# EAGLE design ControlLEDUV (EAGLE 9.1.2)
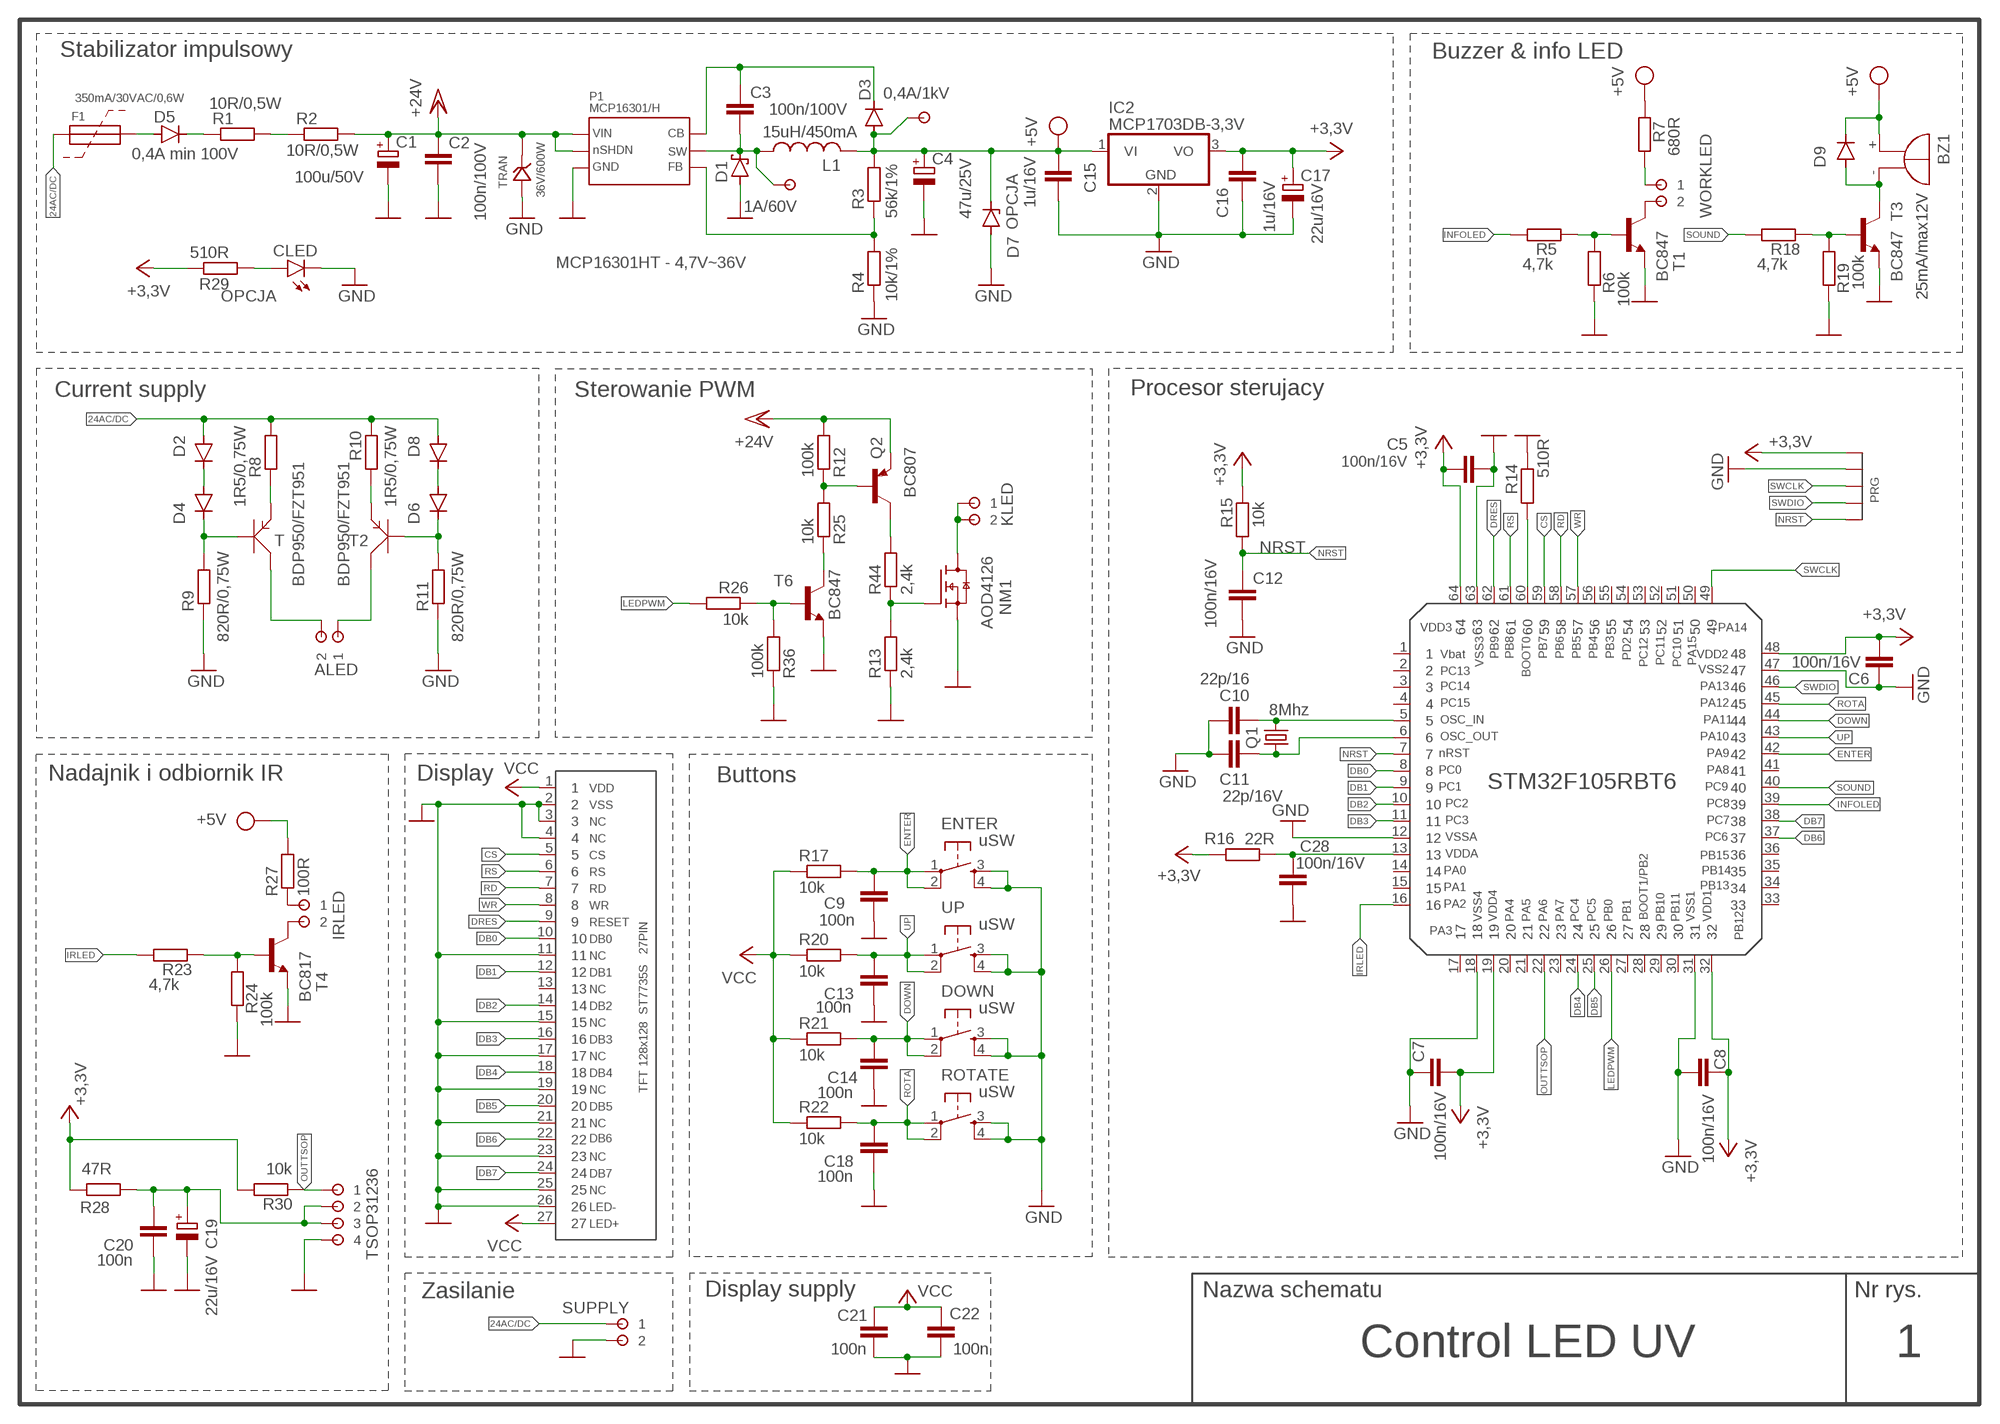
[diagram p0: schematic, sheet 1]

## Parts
ALED  ARK254  [ARK254]
BZ1  25mA/max12V  F/TMB  [F/TMB]
C1  100u/50V  CPOL-EU175TMP-0810  [175TMP-0810]
C2  100n/100V  C-EUC1206  [C1206]
C3  100n/100V  C-EUC0805  [C0805]
C4  47u/25V  CPOL-EU153CLV-0605  [153CLV-0605]
C5  100n/16V  C-EUC0805  [C0805]
C6  100n/16V  C-EUC0805  [C0805]
C7  100n/16V  C-EUC0805  [C0805]
C8  100n/16V  C-EUC0805  [C0805]
C9  100n  C-EUC0805  [C0805]
C10  22p/16  C-EUC0805  [C0805]
C11  22p/16V  C-EUC0805  [C0805]
C12  100n/16V  C-EUC0805  [C0805]
C13  100n  C-EUC0805  [C0805]
C14  100n  C-EUC0805  [C0805]
C15  1u/16V  C-EUC0805  [C0805]
C16  1u/16V  C-EUC0805  [C0805]
C17  22u/16V  CPOL-EU153CLV-0505  [153CLV-0505]
C18  100n  C-EUC0805  [C0805]
C19  22u/16V  CPOL-EU153CLV-0505  [153CLV-0505]
C20  100n  C-EUC0805  [C0805]
C21  100n  C-EUC0805  [C0805]
C22  100n  C-EUC0805  [C0805]
C28  100n/16V  C-EUC0805  [C0805]
CLED  LEDCHIPLED_0805  [CHIPLED_0805]
D1  1A/60V  SCHOTTKY-DIODESMD  [SMB]
D2  DIODE-MINIMELF  [MINIMELF]
D3  0,4A/1kV  DIODE-MINIMELF  [MINIMELF]
D4  DIODE-MINIMELF  [MINIMELF]
D5  0,4A min 100V  DIODE-MINIMELF  [MINIMELF]
D6  DIODE-MINIMELF  [MINIMELF]
D7  ZENER-DIODESOD80C  [SOD80C]
D8  DIODE-MINIMELF  [MINIMELF]
D9  DIODE-MINIMELF  [MINIMELF]
DOWN  uSW  DTSM-6  [DTSM-6]
ENTER  uSW  DTSM-6  [DTSM-6]
F1  350mA/30VAC/0,6W  FUSE1  [FUSE1]
IC2  MCP1703DB-3,3V  MCP1703DB  [SOT223]
IRLED  ARK254  [ARK254]
KLED  ARK254  [ARK254]
L1  15uH/450mA  L-USL4532P  [L4532P]
NM1  AOD4126  [AOD4126]
P1  MCP16301/H  MCP16301  [MCP16301]
PRG  GOLDPIN5  [GOLDPIN5]
Q1  8Mhz  CRYSTALHC49S  [HC49/S]
Q2  BC807  BC807-16LT1SMD  [SOT23-BEC]
R1  10R/0,5W  R-EU_M1206  [M1206]
R2  10R/0,5W  R-EU_M1206  [M1206]
R3  56k/1%  R-EU_R0805  [R0805]
R4  10k/1%  R-EU_R0805  [R0805]
R5  4,7k  R-EU_R0805  [R0805]
R6  100k  R-EU_R0805  [R0805]
R7  680R  R-EU_R0805  [R0805]
R8  1R5/0,75W  R-EU_R2010  [R2010]
R9  820R/0,75W  R-EU_R2010  [R2010]
R10  1R5/0,75W  R-EU_R2010  [R2010]
R11  820R/0,75W  R-EU_R2010  [R2010]
R12  100k  R-EU_R0805  [R0805]
R13  2,4k  R-EU_R0805  [R0805]
R14  510R  R-EU_R0805  [R0805]
R15  10k  R-EU_R0805  [R0805]
R16  22R  R-EU_R0805  [R0805]
R17  10k  R-EU_R0805  [R0805]
R18  4,7k  R-EU_R0805  [R0805]
R19  100k  R-EU_R0805  [R0805]
R20  10k  R-EU_R0805  [R0805]
R21  10k  R-EU_R0805  [R0805]
R22  10k  R-EU_R0805  [R0805]
R23  4,7k  R-EU_R0805  [R0805]
R24  100k  R-EU_R0805  [R0805]
R25  10k  R-EU_R0805  [R0805]
R26  10k  R-EU_R0805  [R0805]
R27  100R  R-EU_M1206  [M1206]
R28  47R  R-EU_R0805  [R0805]
R29  510R  R-EU_R0805  [R0805]
R30  10k  R-EU_R0805  [R0805]
R36  100k  R-EU_R0805  [R0805]
R44  2,4k  R-EU_R0805  [R0805]
ROTATE  uSW  DTSM-6  [DTSM-6]
SUPPLY  ARK254  [ARK254]
T  BDP950/FZT951  BDP950  [FZT951]
T1  BC847  [SOT23]
T2  BDP950/FZT951  BDP950  [FZT951]
T3  BC847  [SOT23]
T4  BC817  BC847  [SOT23]
T6  BC847  [SOT23]
TRAN  36V/600W  TRANSIL2  [DO214AC_BIG]
TSOP31236  ARK254-4  [ARK254-4]
U$3  STM32F105RBT6  [STM32F105RBT6]
U$4  TFT128128  [TFT128128]
U$5  PAD5  [PAD5]
U$6  PAD5  [PAD5]
UP  uSW  DTSM-6  [DTSM-6]
WORKLED  ARK254  [ARK254]

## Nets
24AC/DC: D2.A D8.A F1.1 R8.2 R10.2 SUPPLY.1
CS: U$3.59 U$4.5
DB0: U$3.8 U$4.10
DB1: U$3.9 U$4.12
DB2: U$3.10 U$4.14
DB3: U$3.11 U$4.16
DB4: U$3.24 U$4.18
DB5: U$3.25 U$4.20
DB6: U$3.37 U$4.22
DB7: U$3.38 U$4.24
DOWN: C14.1 DOWN.1 DOWN.2 R21.2 U$3.44
DRES: U$3.62 U$4.9
ENTER: C9.1 ENTER.1 ENTER.2 R17.2 U$3.42
GND: C1.- C2.2 C4.- C5.1 C6.1 C7.1 C8.2 C9.2 C10.1 C11.1 C12.2 C13.2 C14.2 C15.2 C16.2 C17.- C18.2 C19.- C20.2 C21.2 C22.2 C28.1 CLED.C D1.A D7.A DOWN.3 DOWN.4 ENTER.3 ENTER.4 IC2.2(GND) NM1.S P1.2 PRG.2 R4.1 R6.1 R9.1 R11.1 R13.1 R14.2 R19.1 R24.1 R36.1 ROTATE.3 ROTATE.4 SUPPLY.2 T1.2(E) T3.2(E) T4.2(E) T6.2(E) TRAN.P$1 TSOP31236.4 U$3.12 U$3.18 U$3.31 U$3.47 U$3.63 U$4.2 U$4.3 U$4.4 U$4.11 U$4.15 U$4.17 U$4.19 U$4.21 U$4.23 U$4.25 U$4.26 UP.3 UP.4
INFOLED: R5.1 U$3.39
IRLED: R23.1 U$3.16
LAMP1_PWM: Q2.C R44.2
LEDPWM: R26.2 U$3.26
N$1: D5.C R1.1
N$2: R1.2 R2.1
N$3: R5.2 R6.2 T1.1(B)
N$4: T1.3(C) WORKLED.2
N$5: C3.1 D3.C P1.1
N$6: C3.2 D1.C L1.1 P1.6 U$5.1
N$7: P1.3 R3.1 R4.2
N$8: R7.1 WORKLED.1
N$9: D5.A F1.2
N$10: KLED.1 KLED.2 NM1.D
N$11: R8.1 T.3
N$12: ALED.2 T.2 T.4
N$13: D2.C D4.A
N$14: D4.C R9.2 T.1
N$15: ALED.1 T2.2 T2.4
N$16: R10.1 T2.3
N$17: D6.C R11.2 T2.1
N$18: D6.A D8.C
N$19: NM1.G R13.2 R44.1
N$20: C10.2 Q1.2 U$3.5
N$21: C11.2 Q1.1 U$3.6
N$22: R18.2 R19.2 T3.1(B)
N$23: R14.1 U$3.60
N$24: BZ1.- D9.A T3.3(C)
N$25: C28.2 R16.1 U$3.13
N$26: R23.2 R24.2 T4.1(B)
N$27: IRLED.2 T4.3(C)
N$28: Q2.B R12.1 R25.2
N$29: R25.1 T6.3(C)
N$30: R26.1 R36.2 T6.1(B)
N$31: IRLED.1 R27.1
N$32: CLED.A R29.1
N$34: C19.+ C20.1 R28.2 TSOP31236.2 TSOP31236.3
NRST: C12.1 PRG.5 R15.1 U$3.7
OUTTSOP: R30.2 TSOP31236.1 U$3.22
RD: U$3.58 U$4.7
ROTA: C18.1 R22.2 ROTATE.1 ROTATE.2 U$3.45
RS: U$3.61 U$4.6
SOUND: R18.1 U$3.40
SWCLK: PRG.3 U$3.49
SWDIO: PRG.4 U$3.46
UP: C13.1 R20.2 U$3.43 UP.1 UP.2
VCC: C5.2 C6.2 C7.2 C8.1 C16.1 C17.+ C21.1 C22.1 IC2.3(VO) PRG.1 R15.2 R16.2 R17.1 R20.1 R21.1 R22.1 R28.1 R29.2 R30.1 U$3.19 U$3.32 U$3.48 U$3.64 U$4.1 U$4.27 ; supply symbol labelled +3,3V
VCC/2: C1.+ C2.1 P1.4 P1.5 Q2.E R2.2 R12.2 TRAN.P$2 ; supply symbol labelled +24V
VDD: BZ1.+ C4.+ C15.1 D3.A D7.C D9.C IC2.1(VI) L1.2 R3.2 R7.2 R27.2 U$6.1 ; supply symbol labelled +5V
WR: U$3.57 U$4.8
Unconnected: U$3.1 U$3.2 U$3.3 U$3.4 U$3.14 U$3.15 U$3.17 U$3.20 U$3.21 U$3.23 U$3.27 U$3.28 U$3.29 U$3.30 U$3.33 U$3.34 U$3.35 U$3.36 U$3.41 U$3.50 U$3.51 U$3.52 U$3.53 U$3.54 U$3.55 U$3.56 U$4.13

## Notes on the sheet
- Stabilizator impulsowy | Buzzer & info LED
- OPCJA
- MCP16301HT - 4,7V~36V
- OPCJA
- Current supply | Sterowanie PWM | Procesor sterujacy
- Nadajnik i odbiornik IR | Display | Buttons
- Zasilanie | Display supply
- Control LED UV | 1

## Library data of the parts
ALED IRLED KLED SUPPLY WORKLED = ark254:ARK254
BZ1 = buzzer:F/TMB: BUZZER; OC_FARNELL: unknown; OC_NEWARK: unknown
C1 C4 C17 C19 = rcl:CPOL-EU: POLARIZED CAPACITOR, European symbol; SPICEPREFIX: C
C2 C3 C5-C16 C18 C20-C22 C28 = rcl:C-EU: CAPACITOR, European symbol; SPICEPREFIX: C
CLED = led:LED: LED
D1 = diode:SCHOTTKY-DIODE: Schottky Diode
D2-D6 D8 D9 = diode:DIODE-: DIODE
D7 = diode:ZENER-DIODE: Z-Diode
DOWN ENTER ROTATE UP = switch-tact:DTSM-6
F1 = Fuse:FUSE1
IC2 = linear:MCP1703: 250 mA, 16V, Low Quiescent Current LDO Regulator Source: http://ww1.microchip.com/downloads/en/DeviceDoc/22049b.pdf
L1 = rcl:L-US: INDUCTOR, American symbol; SPICEPREFIX: L
NM1 = AOD4126:AOD4126
P1 = Regulatory:MCP16301
PRG = Goldpin5:GOLDPIN5: 3 Goldpin
Q1 = crystal:CRYSTAL: CRYSTAL; OC_FARNELL: 1667008; OC_NEWARK: unknown
Q2 = transistor-pnp:BC807*: PNP Transistror
R1-R30 R36 R44 = rcl:R-EU_: RESISTOR, European symbol; SPICEPREFIX: R
T T2 = transistorpnp:BDP950
T1 T3 T4 = transistor-neu-to92:BC847: NPN TRANSISTOR
T6 = transistor:BC847: NPN TRANSISTOR; SPICEPREFIX: J
TRAN = transil2:TRANSIL2
TSOP31236 = ark254:ARK254-4
U$3 = STM32F105RBT6:STM32F105RBT6
U$4 = tft128128:TFT128128
U$5 U$6 = PAD:PAD5

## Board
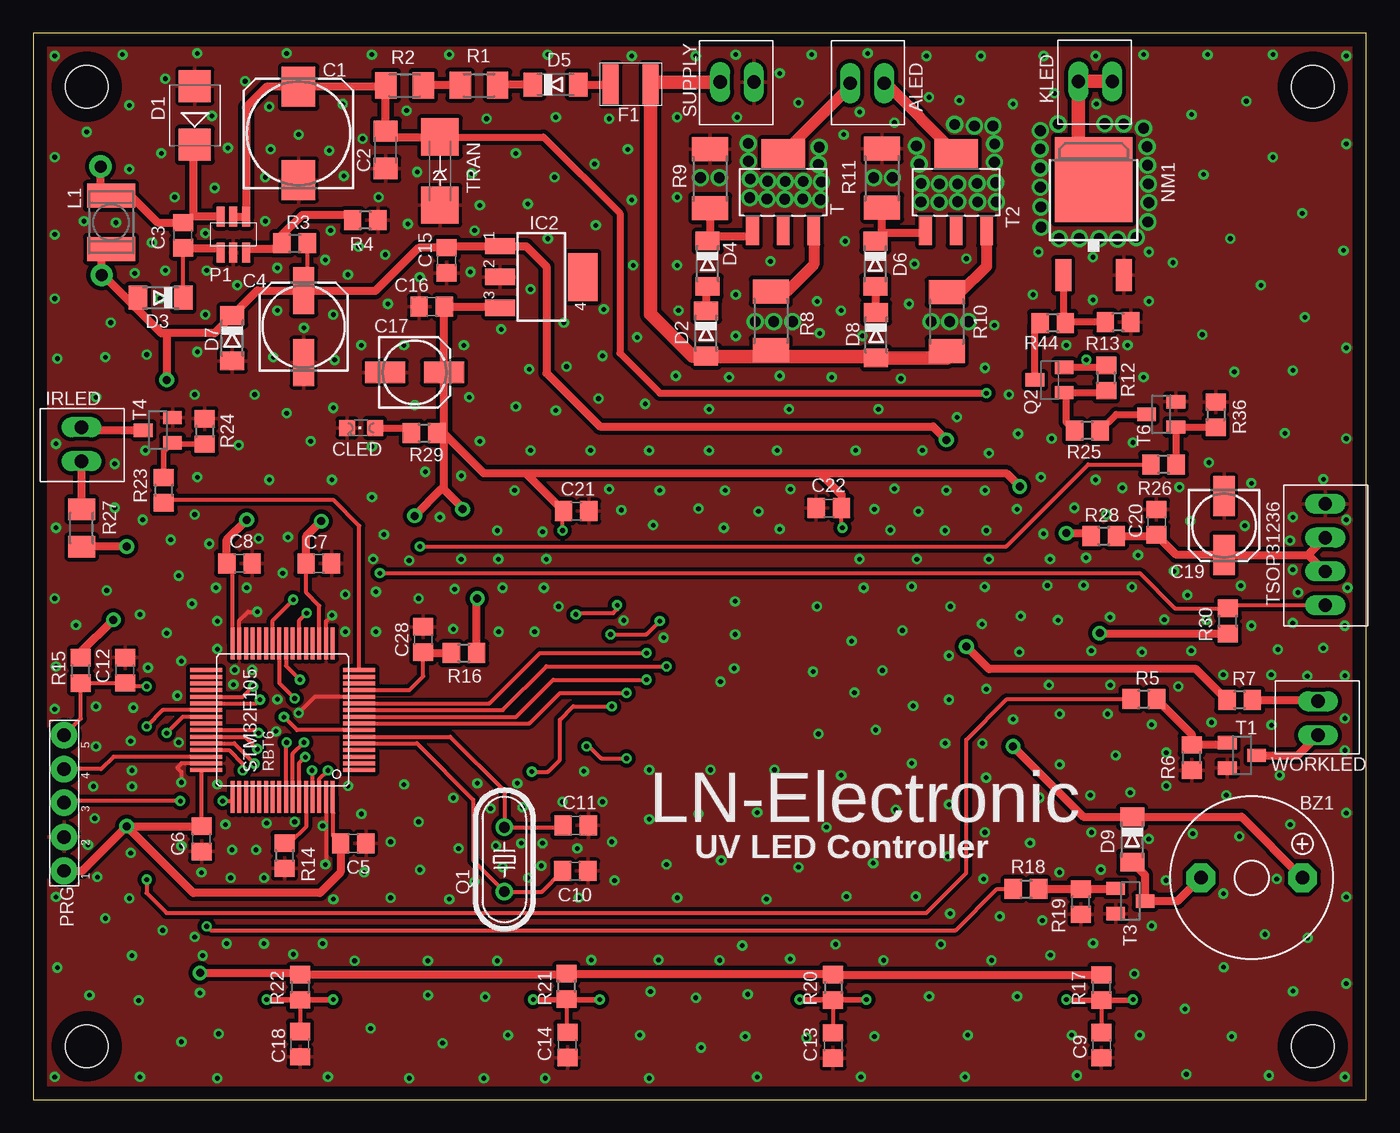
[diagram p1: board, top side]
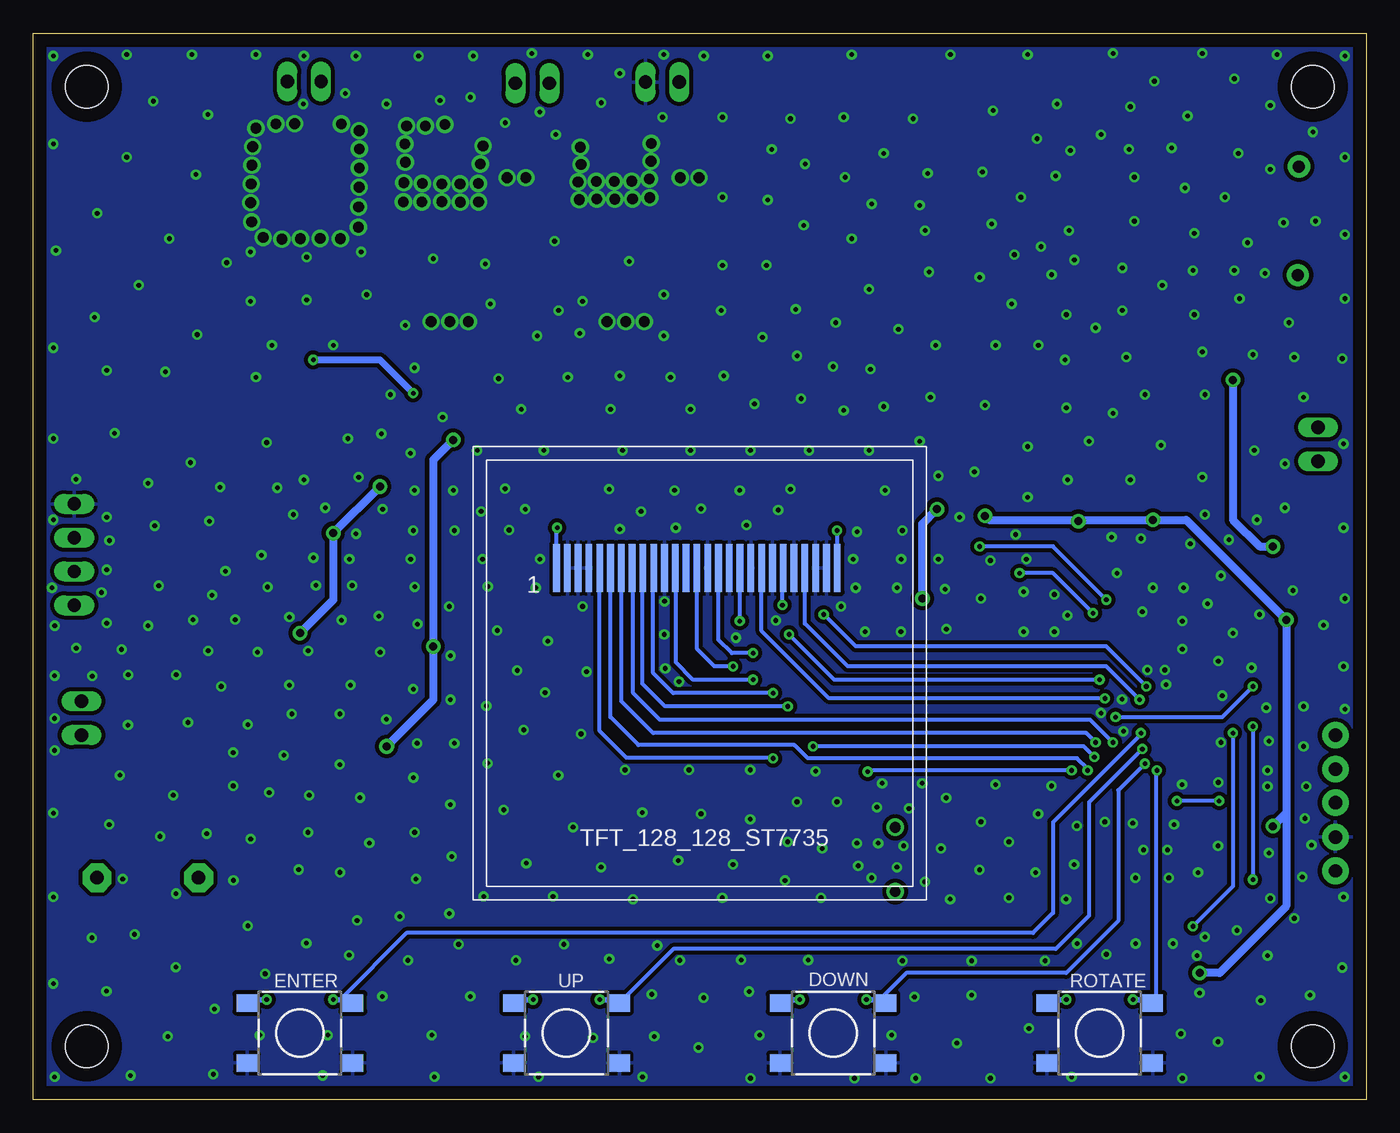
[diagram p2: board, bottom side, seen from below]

Size 100 x 80 mm. Coordinates in mm from the lower left corner, seen from the top.
Outline: 0,0 100,0 100,80 0,80 0,0
Copper layers (1*16): Top 0.035mm / dielectric 1.5mm / Bottom 0.035mm
Design rules "default *": minimum track width 6mil, minimum drill 0.35mm, track to track 6mil, track to pad 6mil, pad to pad 6mil, via to via 6mil, smd to smd 6mil, copper to edge 40mil, drill to drill 6mil, minimum pad ring 10mil, minimum via ring 8mil, stop-mask expansion 4mil, vias tented up to drill 40mil, thermal gap 10mil
Holes 3.2 mm at 4,4 96,4 96,76 4,76

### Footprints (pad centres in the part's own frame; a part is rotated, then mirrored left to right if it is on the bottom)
ARK254 = drill 1 long: 1 -0.06,0; 2 2.48,0
F/TMB = drill 1.016 pad 2.159 octagon: + 3.81,0; - -3.81,0
175TMP-0810 = smd 3 x 2.5: + 3.5,0; - -3.5,0
C1206 = smd 1.6 x 1.8: 1 -1.4,0; 2 1.4,0
C0805 = smd 1.3 x 1.5: 1 -0.95,0; 2 0.95,0
153CLV-0605 = smd 3.5 x 1.6: + 2.7,0; - -2.7,0
153CLV-0505 = smd 3 x 1.6: + 2.2,0; - -2.2,0
CHIPLED_0805 = smd 1.2 x 1.2: A 0,-1.05; C 0,1.05
SMB = smd 2.4 x 2.4: A 2.2,0; C -2.2,0
MINIMELF = smd 1.4 x 1.8: A 1.7,0; C -1.7,0
SOD80C = smd 1.4 x 1.8: A 1.7,0; C -1.7,0
DTSM-6 = smd 1.55 x 1.3: 1 -3.975,2.25; 2 3.975,2.25; 3 -3.975,-2.25; 4 3.975,-2.25
FUSE1 = smd 1.2 x 3: 1 -0.5,0; 2 2.5,0
SOT223 = smd 1.219 x 2.235: 1 -2.311,-3.099; 2 0,-3.099; 3 2.311,-3.099 | smd 3.6 x 2.2: 4 0,3.099
L4532P = smd 1.8 x 3.6: 1 -2,0; 2 2,0
AOD4126 = smd 5.8 x 6.4: D 0,1.103 | smd 1.2 x 2.4: G -2.28,-6.07; S 2.28,-6.07
MCP16301 = smd 0.6 x 1.5: 1 0,0; 2 0.95,0; 3 1.9,0; 4 1.9,2.7; 5 0.95,2.7; 6 0,2.7
GOLDPIN5 = drill 1 pad 2: 1 0,0.01; 2 2.54,0.01; 3 5.12,0.01; 4 7.64,0.01; 5 10.18,0.01
HC49/S = drill 0.813: 1 -2.413,0; 2 2.413,0
SOT23-BEC = smd 1 x 1.4: B -0.95,-1.1; C 0,1.1; E 0.95,-1.1
M1206 = smd 1.6 x 2: 1 -1.4,0; 2 1.4,0
R0805 = smd 1.3 x 1.5: 1 -0.95,0; 2 0.95,0
R2010 = smd 1.8 x 2.7: 1 -2.2,0; 2 2.2,0
FZT951 = smd 0.95 x 2.15: 1 -2.3,-2.9; 2 0,-2.9; 3 2.3,-2.9 | smd 3.25 x 2.15: 4 0,2.9
SOT23 = smd 1 x 1.4: 1 -0.95,-1.1; 2 0.95,-1.1; 3 0,1.1
DO214AC_BIG = smd 2.8 x 2.8: P$1 -2.558,0; P$2 2.558,0
ARK254-4 = drill 1 long: 1 -0.06,0; 2 2.48,0; 3 5.02,0; 4 7.56,0
STM32F105RBT6 = smd 0.3 x 2.4: 1 0,0; 2 0.5,0; 3 1,0; 4 1.5,0; 5 2,0; 6 2.5,0; 7 3,0; 8 3.5,0; 9 4,0; 10 4.5,0; 11 5,0; 12 5.5,0; 13 6,0; 14 6.5,0; 15 7,0; 16 7.5,0; 33 7.5,11.5; 34 7,11.5; 35 6.5,11.5; 36 6,11.5; 37 5.5,11.5; 38 5,11.5; 39 4.5,11.5; 40 4,11.5; 41 3.5,11.5; 42 3,11.5; 43 2.5,11.5; 44 2,11.5; 45 1.5,11.5; 46 1,11.5; 47 0.5,11.5; 48 0,11.5 | smd 2.4 x 0.3: 17 9.5,2; 18 9.5,2.5; 19 9.5,3; 20 9.5,3.5; 21 9.5,4; 22 9.5,4.5; 23 9.5,5; 24 9.5,5.5; 25 9.5,6; 26 9.5,6.5; 27 9.5,7; 28 9.5,7.5; 29 9.5,8; 30 9.5,8.5; 31 9.5,9; 32 9.5,9.5; 49 -2,9.5; 50 -2,9; 51 -2,8.5; 52 -2,8; 53 -2,7.5; 54 -2,7; 55 -2,6.5; 56 -2,6; 57 -2,5.5; 58 -2,5; 59 -2,4.5; 60 -2,4; 61 -2,3.5; 62 -2,3; 63 -2,2.5; 64 -2,2
TFT128128 = smd 0.5 x 3.6: 1 -0.746,-0.127; 2 0.064,-0.127; 3 0.874,-0.127; 4 1.684,-0.127; 5 2.494,-0.127; 6 3.304,-0.127; 7 4.114,-0.127; 8 4.924,-0.127; 9 5.734,-0.127; 10 6.544,-0.127; 11 7.354,-0.127; 12 8.164,-0.127; 13 8.974,-0.127; 14 9.784,-0.127; 15 10.594,-0.127; 16 11.404,-0.127; 17 12.214,-0.127; 18 13.024,-0.127; 19 13.834,-0.127; 20 14.644,-0.127; 21 15.454,-0.127; 22 16.264,-0.127; 23 17.074,-0.127; 24 17.884,-0.127; 25 18.694,-0.127; 26 19.504,-0.127; 27 20.314,-0.127
PAD5 = drill 0.9 pad 1.676: 1 0,0

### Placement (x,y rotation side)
ALED  63.77,76.25 180 top
BZ1  91.41,16.64 0 top
C1  19.9,72.49 90 top
C2  26.44,71.25 270 top
C3  11.24,64.85 90 top
C4  20.28,58 90 top
C5  24,19.22 180 top
C6  12.61,19.55 90 top
C7  21.42,40.22 180 top
C8  15.47,40.22 0 top
C9  80.14,4.08 270 top
C10  40.66,17.15 180 top
C11  40.69,20.57 180 top
C12  6.88,32.21 90 top
C13  60.01,4.06 270 top
C14  40.08,4.1 270 top
C15  31.01,62.97 270 top
C16  29.89,59.49 180 top
C17  28.61,54.56 0 top
C18  20.01,4.16 270 top
C19  89.34,43.07 270 top
C20  84.27,43.31 90 top
C21  40.74,44.14 0 top
C22  59.69,44.37 180 top
C28  29.26,34.52 270 top
CLED  24.59,50.39 90 top
D1  12.12,73.83 90 top
D2  50.48,57.48 270 top
D3  9.55,60.16 180 top
D4  50.6,62.71 270 top
D5  39.19,76.16 0 top
D6  63.17,62.71 270 top
D7  14.92,57.12 270 top
D8  63.23,57.35 270 top
D9  82.45,19.51 270 top
DOWN  40,5 0 bottom
ENTER  80,5 0 bottom
F1  45.81,76.18 180 top
IC2  38.12,61.72 270 top
IRLED  3.61,47.96 90 top
KLED  78.47,76.39 0 top
L1  5.83,65.81 270 top
NM1  79.55,67.91 0 top
P1  14.05,63.56 0 top
PRG  2.32,17.15 90 top
Q1  35.34,18.01 270 top
Q2  76.25,53.99 90 top
R1  33.43,76.1 180 top
R2  27.86,76.09 180 top
R3  19.61,64.25 0 top
R4  24.9,65.97 180 top
R5  83.31,30.05 0 top
R6  86.9,25.66 90 top
R7  90.51,29.98 180 top
R8  55.33,58.43 270 top
R9  50.77,69.1 270 top
R10  68.53,58.37 270 top
R11  63.67,69.13 270 top
R12  80.49,54.14 90 top
R13  81.39,58.32 180 top
R14  18.84,18.3 270 top
R15  3.57,32.19 90 top
R16  32.3,33.51 0 top
R17  80.14,8.41 270 top
R18  74.47,15.8 0 top
R19  78.6,14.84 90 top
R20  60.01,8.42 270 top
R21  39.99,8.5 270 top
R22  20.01,8.43 270 top
R23  9.8,45.72 90 top
R24  12.86,50.13 270 top
R25  79.08,50.18 180 top
R26  84.79,47.65 180 top
R27  3.63,42.88 270 top
R28  80.3,42.29 0 top
R29  29.32,50.01 0 top
R30  89.63,35.9 90 top
R36  88.71,51.38 270 top
R44  76.48,58.26 180 top
ROTATE  20,5 0 bottom
SUPPLY  51.59,76.35 0 top
T  56.26,68.08 0 top
T1  90.69,25.82 270 top
T2  69.23,68.08 0 top
T3  82.31,14.89 270 top
T4  9.34,50.22 90 top
T6  84.62,51.41 90 top
TRAN  30.51,69.67 90 top
TSOP31236  96.93,37.14 90 top
U$3  24.46,24.72 90 top
U$4  60,40 0 bottom
U$5  5.04,70.01 0 top
U$6  5.13,61.86 0 top
UP  60,5 0 bottom
WORKLED  96.39,29.82 270 top

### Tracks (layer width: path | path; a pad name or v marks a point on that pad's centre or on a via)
24AC/DC
  Top 0.3: 46.48,76.35 F1.1 | D2.A 51,55.78 | 56.03,55.74 55.54,56.23 R8.2 55.81,55.75 | 68.53,55.65 R10.2
  Top 1.016: SUPPLY.1 46.48,76.35 | 56.03,55.74 51.04,55.74 51,55.78 49.47,55.78 46.31,58.94 F1.1 | 55.81,55.75 63.13,55.75 D8.A 68.53,55.65
CS  (via drill 0.35)
  Top 0.3: U$3.59 19.96,25.26 v20.4,25.7 | v44.5,25.6 42.6,25.6 41.7,26.5 v41.5,26.5
  Bottom 0.3: v20.4,25.7 21.2,26.5 v41.5,26.5 | U$4.5 57.51,27.64 55.51,25.65 44.55,25.65 v44.5,25.6
DB0  (via drill 0.35)
  Top 0.3: U$3.8 37.22,28.22 39.5,30.5 v44.5,30.5
  Bottom 0.3: v44.5,30.5 52,30.5 53.5,32 53.5,39.83 U$4.10
DB1  (via drill 0.35)
  Top 0.3: U$3.9 36.22,28.72 39,31.5 v46,31.5
  Bottom 0.3: v46,31.5 50.5,31.5 51.8,32.8 51.8,39.84 U$4.12
DB2  (via drill 0.35)
  Top 0.3: U$3.10 35.22,29.22 38.5,32.5 v47.5,32.5
  Bottom 0.3: v47.5,32.5 48.9,32.5 50.2,33.8 50.2,39.86 U$4.14
DB3  (via drill 0.35)
  Top 0.3: U$3.11 34.22,29.72 38,33.5 v46,33.5
  Bottom 0.3: v46,33.5 47.6,33.5 48.6,34.5 U$4.16
DB4  (via drill 0.35)
  Top 0.3: U$3.24 18.96,32.54 v20,31.5 | v43.3,34.9 46,34.9 v47,35.9
  Bottom 0.3: v20,31.5 39.9,31.5 v43.3,34.9 | v47,35.9 46.98,35.92 U$4.18
DB5  (via drill 0.35)
  Top 0.3: U$3.25 18.46,31.24 v19.6,30.1
  Bottom 0.3: v19.6,30.1 40.3,30.1 45.36,35.16 U$4.20
DB6  (via drill 0.35)
  Top 0.3: U$3.37 15.72,30.22 v16.5,31 | v43.8,37.1 43.8,36.8 43.5,36.5 40.8,36.5 v40.7,36.4
  Bottom 0.3: v16.5,31 19.5,34 38.3,34 v40.7,36.4 | v43.8,37.1 43.8,39.81 U$4.22
DB7  (via drill 0.35)
  Top 0.3: U$3.38 16.72,29.72 v17,30
  Bottom 0.3: v17,30 19.5,32.5 38.9,32.5 42.12,35.72 U$4.24
DOWN  (via drill 0.35)
  Top 0.3: R21.2 40.04,7.5 | R21.2 39.94,7.5 | R21.2 39.99,5.13 C14.1 | U$3.44 15.08,26.72 v16.6,25.2
  Top 0.406: 40.04,7.5 v42.5,7.5 | 39.94,7.5 v37.5,7.5
  Bottom 0.3: 43.73,7.5 DOWN.1 | 36.27,7.5 36.14,7.36 | 36.14,7.36 DOWN.2 | v16.6,25.2 18.6,23.2 18.6,13.4 22.5,9.5 34.5,9.5 36.14,7.86 36.14,7.36
  Bottom 0.406: v42.5,7.5 43.73,7.5 | v37.5,7.5 36.27,7.5
DRES  (via drill 0.35)
  Top 0.3: U$3.62 21.46,24.06 v22.1,24.7 | v37.4,24.6 38.6,24.6 39.5,25.5 39.5,28.5 40.5,29.5 v43.4,29.5
  Bottom 0.3: v22.1,24.7 37.3,24.7 v37.4,24.6 | v43.4,29.5 52.6,29.5 54.3,31.2 54.3,39.84 U$4.9
ENTER  (via drill 0.35)
  Top 0.3: 77.54,7.46 v77.5,7.5 | 82.46,7.46 v82.5,7.5 | R17.2 C9.1 | U$3.42 16.58,27.72 16.8,27.5 v16.9,27.5
  Top 0.406: 77.54,7.46 R17.2 82.46,7.46
  Bottom 0.3: ENTER.2 76.28,7.5 77,7.5 72,12.5 25,12.5 23.5,14 23.5,20.8 16.9,27.4 v16.9,27.5 | 83.72,7.5 ENTER.1
  Bottom 0.406: v77.5,7.5 77,7.5 | v82.5,7.5 83.72,7.5
GND  (via drill 0.35, 0.8 pad 1.3)
  Top 0.3: U$3.12 21.12,30.22 v19.9,29 | U$3.18 21.96,35.88 v22.41,36.33 | U$3.31 15.46,35.96 16.1,36.6 v16.8,36.6 | U$3.47 11.12,25.22 10.8,24.9 11.1,24.6 v11.1,23.8 | U$3.63 21.96,17.68 v21.91,17.63
  other vias: 1.6,78.3 1.6,70.7 1.6,64.9 1.6,60.1 1.8,55.6 1.7,49.2 1.7,42.9 1.6,37.6 1.7,32.5 1.6,29.3 1.7,15.2 1.8,9.9 1.6,1.7 8,1.7 13.8,1.6 22.1,1.7 28.2,1.6 33.8,1.6 38.4,1.6 46.2,1.6 54.3,1.7 62.1,1.7 69.9,1.7 78.3,1.8 86.5,1.9 98.4,1.7 98.5,8.7 98.5,15.2 98.5,21.5 98.4,26.2 98.4,31.8 98.6,38.4 98.5,43.5 98.5,49.6 98.5,56.4 98.3,63.7 98.5,71.7 98.5,78.3 93,78.4 88.1,78.4 83.3,78.4 75.8,78.3 71.1,78.3 67,78.3 62.6,78.5 58.4,78.4 49.7,78.3 44.9,78.3 38.6,78.4 31.2,78.4 25.4,78.4 19,78.5 12.3,78.5 6.7,78.4 7.2,74.6 4,72.6 7.2,69.8 10.6,67.7 9.6,71 9.9,76.6 13.4,73.8 15.9,76.4 17.7,74.5 17.4,69.2 19.9,72.4 23.2,74.7 23.3,69.3 24.7,72.1 28,74.2 17.4,65.9 25.9,67.7 28.8,69.6 32.9,69.5 36.2,71 39.1,69.2 33.5,67.1 37.1,67.2 42.2,65.6 34,73.6 39.2,73.7 44.6,71.3 44.9,67.5 42.1,70.2 48.3,73.7 52.8,73.7 57.4,74.8 48.3,67.7 82.5,49.3 76.4,49.6 60.8,72.4 64.6,73.3 60.9,64.4 60.6,59.2 58.8,59.9 52.7,60.4 55.3,62.9 48.3,62.6 48.4,59.2 52.7,57.3 62.2,57.3 65.7,59.7 66.1,62.7 62,74.1 70,63.1 73.2,52.9 67.2,75.2 69.48,74.97 73.5,74.7 76.6,75.5 79.75,74.7 75.4,63.6 75,60.4 72.1,58.1 71.4,54.9 65.1,54.1 59.9,54.2 56,54.3 52.2,54.2 48.2,54.3 45.3,57.2 45,62.6 59,57.5 86.9,73.9 93,70.7 95.2,66.5 87.8,69.4 85.5,62.8 92.1,61.1 94.5,54.7 87.7,57.4 83.3,54.2 93.9,50 79.5,60 79.5,63.2 88.2,47.8 94.5,43.7 86.8,43.4 95.4,58.7 90.1,54.6 89.8,64.6 91,74.9 69.3,51.2 75.6,46.7 71.7,48.5 78.1,44.4 81.7,45.9 39.8,58.3 42.7,55.8 42.4,52.6 45.9,52.2 42.8,59.3 50.7,51.8 56.7,51.8 63.4,51.8 66.7,48.7 61.7,48.7 55.8,48.7 50.7,48.7 46.2,48.7 41.8,48.7 37.3,48.7 33.5,49.4 32.7,52.7 32.3,56.6 35.1,57.8 37.3,60.8 37.2,54.8 39.2,51.7 36.2,52 29,61.7 32.8,62.1 26.6,59.7 22.5,58.9 22.6,55.5 27.8,56.6 22.5,51.9 28.6,52.1 18.3,59.2 18,55.7 12.3,56.1 12.1,52.9 16.6,52.9 15.4,49.1 12.3,46.7 17.7,46.5 22.4,46.5 25.4,45.2 29.4,47.1 25.4,49 20.8,49.4 19,51.5 18.3,62.4 15.3,61.1 12.9,58.9 13,62.2 9.9,62.2 7.6,62 8.9,64.3 6.2,65.8 3.8,65.9 9.5,60.1 13.6,68.4 14.6,71.4 52.7,78.4 79.7,78.3 24.6,56.6 4.7,52.7 8.5,55.9 5.8,58.3 6.1,47.7 8.4,48.7 6.1,44.4 8.2,43.5 5.5,38.2 10.3,42 12.1,43.9 3.2,35.6 5.4,55.7 12.9,65 21.9,63 22.3,65.2 23.6,61.9 26.4,63.4 24.4,64 28.1,65.7 33.1,65.2 38.6,64.6 20.3,57.9 40,55 43.2,73.6 73.8,44.3 71.5,42.7 71.4,45.7 68.5,45.7 68.4,42.7 63.1,44.3 56.8,45.8 56,42.8 51.8,42.9 51.9,45.7 47,45.7 46.5,43.1 43.2,45.8 30.5,43.7 26.3,42.4 32.1,46.8 36.1,45.7 38.2,42.6 34.8,42.7 13.2,41.7 10.9,39.3 8,36.4 16,38.4 16.9,42.1 19.1,42.2 18.7,39.5 23.4,37.9 23.4,35.1 25.7,38.1 31.6,38.3 25.7,35.1 31.5,35.3 28.9,37.6 35.2,38.4 38.3,38.4 39.4,37 37.6,35.1 34.9,35.1 13.7,38.4 13.8,35.9 13.8,33.8 11.1,32.9 10.8,30.3 8.6,32.4 10,35 11.9,37.2 7.5,29.4 4.7,29.5 4.7,26.5 7.3,26.9 4.5,23.5 7.4,24.7 7.4,23.5 10.9,26.8 4.6,21.1 4.1,19.1 4.8,16.7 5.4,13.6 7.2,15.1 7.3,18.5 9.7,12.7 12.7,10.8 14.5,11.7 17.3,11.7 19.5,10.9 21.7,11.7 24.1,10.4 29.6,10.4 34.8,10.4 41.86,10.46 46.9,10.47 51.49,10.45 53.19,11.55 56.79,10.55 60.19,11.65 63.79,10.45 68.09,11.65 71.89,10.45 68.79,13.95 71.29,16.55 71.39,20.05 71.49,24.15 75.49,22.65 79.39,20.05 80.09,17.25 74.79,19.25 76.99,17.05 83.69,19.55 86.99,19.95 90.49,19.75 93.29,16.55 89.29,15.45 84.99,16.45 52.59,32.35 47.29,34.65 44.29,35.95 25.49,40.55 28.19,40.45 32.09,40.55 34.89,40.55 38.49,40.55 61.99,40.55 66.29,40.55 71.69,40.55 75.79,42.45 76.29,40.55 78.99,40.65 82.89,40.85 85.59,39.65 86.59,37.85 90.59,38.55 94.49,39.75 94.89,38.05 90.89,43.05 94.29,41.95 91.39,46.25 85.99,45.95 96.79,46.55 73.89,49.95 98.39,35.55 94.49,35.75 91.39,35.55 88.02,35.99 84.86,36.01 82.43,38.46 78.8,38.58 80.79,36.2 95.58,31.77 92.88,31.87 89.28,31.87 86.88,33.67 96.78,33.87 93.38,33.77 83.18,33.57 79.38,33.67 76.88,35.97 76.08,38.57 71.38,38.47 71.18,35.67 73.98,33.57 74.08,36.27 58.8,37 62.3,38.4 65.9,38.5 68.8,37 68.7,33.3 65.2,35.2 61.4,34.4 58.5,32.1 63.7,32.2 68.7,30 71.5,30.8 76.2,31.1 80.8,31.1 85.9,31 88.4,28.3 92.9,28.1 98.4,28.6 15.11,32.23 16.41,32.23 15.01,31.13 18.31,30.03 18.21,27.63 13.81,23.63 23.61,23.53 27.81,23.63 31.51,22.63 24.61,21.43 26.81,19.33 28.91,20.83 31.91,18.83 24.81,17.03 29.01,17.23 33.11,16.33 31.21,15.03 26.81,15.13 22.51,15.03 17.51,20.73 19.61,20.83 16.71,18.73 17.31,16.63 14.81,16.63 14.91,18.73 14.41,20.63 12.61,17.03 11.11,19.03 7.91,7.43 13.91,4.93 25.31,5.33 29.61,7.83 35.61,4.83 30.71,4.23 45.51,4.83 49.71,7.63 53.41,4.73 58.01,4.63 67.21,7.73 73.81,7.73 63.11,4.73 70.11,4.83 77.91,4.83 83.01,4.83 89.91,4.73 94.51,8.13 95.61,12.13 89.31,9.93 82.61,9.43 83.91,13.03 79.51,11.73 75.71,13.43 72.51,13.73 76.31,10.83 38.21,19.23 36.61,19.23 34.71,19.03 34.31,21.83 36.71,21.93 39.71,22.33 42.71,22.33 43.41,19.33 43.61,16.43 40.91,15.13 35.21,17.43 37.11,16.63 38.11,17.53 40.81,18.83 33.31,23.73 36.31,23.73 41.31,24.63 46.21,24.73 50.81,24.73 55.61,24.73 58.91,27.43 61.61,30.53 66.01,29.53 68.41,26.73 63.21,27.73 65.91,25.23 68.71,22.13 60.61,24.33 64.71,21.73 68.61,18.23 66.21,15.23 63.01,17.73 59.51,20.43 54.31,21.53 57.41,17.43 61.01,15.23 55.01,15.03 51.61,17.93 49.91,21.43 46.21,21.03 47.51,17.63 48.31,15.13 71.21,26.73 73.51,28.53 77.01,28.93 80.61,28.93 83.91,28.13 85.01,26.03 85.01,23.53 82.31,23.03 79.31,22.83 77.01,25.13 81.21,25.83 66.41,44.13 64.61,45.83 64.31,42.73 54.41,44.13 49.91,44.33 44.11,44.23 56,77 79.7,46.5 80.5,43.9 77.5,56.6 82.1,56.6 83.7,59.9 83.7,63.6 92.4,12.4 86.4,6.8 92.7,1.8 50.1,3.9 53.6,7.9 46.3,8.1 33.9,7.7 12.5,8 7.4,10.8 83.69,67.3 75.56,68.46 75.53,69.89 75.53,71.32 75.56,72.69 76.89,73.19 75.59,66.98 75.62,65.46 76.96,64.59 78.48,64.62 79.96,64.59 81.36,64.56 82.76,64.68 83.62,65.84 83.65,68.7 83.6,70.11 83.55,71.49 83.29,72.88 81.81,73.2 80.39,73.22 66.62,68.73 67.98,68.69 66.59,67.35 67.96,67.33 69.34,67.37 69.36,68.71 70.81,68.73 70.85,67.35 72.25,67.35 72.21,68.8 72.1,70.33 72.12,71.71 71.99,73.04 66.46,70.2 66.26,71.54 70.6,73.05 69.12,73.16 58.96,71.46 58.91,70.15 53.78,69.08 55.09,68.91 56.41,68.89 57.77,68.89 59.13,68.84 53.76,67.67 55.04,67.57 56.38,67.56 57.73,67.57 59.05,67.52 53.66,70.41 53.64,71.75 54.16,58.37 55.56,58.37 56.96,58.37 70.16,58.37 68.76,58.37 67.36,58.37 51.46,69.17 50.06,69.17 64.46,69.17 63.06,69.17 21.71,20.53 89.51,22.83 93.51,24.33 94.31,20.63 22.2,71.2 17.8,71.3 52.65,37.38 52.66,34.9 51.56,31.35 11.11,4.33 4.21,7.83 12.1,12.2
  pour Top (isolate 0.305): 0.1,79.8 0.1,0.1 100,0.1 100,79.9 0.1,79.9
  pour Bottom (isolate 0.305): 0.1,79.9 0.1,0.2 100,0.2 100,80 0.1,80
INFOLED  (via drill 0.35)
  Top 0.3: U$3.39 9.72,29.22 v8.5,28 | R5.1 73.05,30.05 70,27 70,17 67,14 10,14 8.5,15.5 v8.5,16.5
  Bottom 0.3: v8.5,28 v8.5,16.5
IRLED
  Top 0.3: U$3.16 24.46,43.04 22.53,44.97 10,44.97 R23.1
LAMP1_PWM
  Top 0.3: 75.15,58.18 75.23,58.26
  Top 0.508: Q2.C 75.15,58.18 | 75.23,58.26 R44.2
LEDPWM  (via drill 0.35)
  Top 0.3: U$3.26 17.96,35.96 v19.5,37.5 | v29,41.5 73,41.5 79.15,47.65 R26.2
  Bottom 0.3: v19.5,37.5 23.5,41.5 v29,41.5
N$1
  Top 0.3: 34.89,76.16 R1.1
  Top 0.61: D5.C 34.89,76.16
N$2
  Top 0.3: R1.2 32.02,76.09
  Top 0.61: 32.02,76.09 R2.1
N$3
  Top 0.3: T1.1 89.42,26.61
  Top 0.61: 89.42,26.61 R6.2 86.9,27.41 R5.2
N$4
  Top 0.61: T1.3 94.87,25.82 WORKLED.2
N$5
  Top 0.3: D3.C 11.25,63.88 C3.1 | 13.71,63.9 P1.1
  Top 0.61: C3.1 13.71,63.9
N$6
  Top 0.3: 12,66.26 11.7,66.26 C3.2 | D1.C 12,71.51 | L1.1 5.04,68.6
  Top 0.61: P1.6 12,66.26 12,71.51 | L1.1 7.32,67.81 9.34,65.8 C3.2 | 5.04,68.6 U$5.1
N$7
  Top 0.3: R3.1 18.46,64.04 18.46,64.24 | 18.46,64.24 18.46,63.86 | R4.2 23.95,66.37 | P1.3 15.95,63.86 | 18.46,64.66 18.46,64.24
  Top 0.61: 15.95,63.86 18.46,63.86 | 23.95,66.37 20.17,66.37 18.46,64.66
N$8
  Top 0.3: 96.29,29.98 WORKLED.1
  Top 0.61: R7.1 96.29,29.98
N$9
  Top 0.3: 43.3,76.16 F1.2
  Top 0.61: D5.A 43.3,76.16
N$10
  Top 0.3: 78.41,70.15 NM1.D
  Top 1.016: KLED.2 KLED.1 78.41,70.15
N$11
  Top 0.813: T.3 58.56,62.66 56.53,60.63 R8.1
N$12
  Top 0.813: T.4 61.28,76 ALED.2
N$13
  Top 0.3: D4.A 50.48,60.9
  Top 0.61: 50.48,60.9 D2.C
N$14
  Top 0.3: 50.77,64.59 D4.C 50.98,64.8 | 54,64.8 54,65.14 T.1
  Top 0.61: R9.2 50.77,64.59 | 50.98,64.8 54,64.8
N$15
  Top 0.3: 63.95,76.25 ALED.1
  Top 0.813: T2.4 63.95,76.25
N$16
  Top 0.3: R10.1 69.57,60.57
  Top 0.813: T2.3 71.53,62.53 69.57,60.57
N$17
  Top 0.3: D6.C 63.67,64.91 63.67,65 | T2.1 66.75,65
  Top 0.61: R11.2 63.67,65 66.75,65
N$18
  Top 0.3: 63.23,60.95 D6.A
  Top 0.61: D8.C 63.23,60.95
N$19
  Top 0.3: 77.27,58.42 R44.1 77.48,58.32
  Top 0.508: NM1.G 77.27,58.42 | R13.2 77.48,58.32
N$20
  Top 0.3: U$3.5 28.78,26.72 33,22.5 33,17.94 Q1.2 38.16,15.6 C10.2
N$21
  Top 0.3: U$3.6 31.28,27.22 35.34,23.16 Q1.1 39.6,20.42 C11.2
N$22
  Top 0.3: R19.2 79,15.79 78.99,15.8 | 81.16,15.79 T3.1
  Top 0.61: 79,15.79 81.16,15.79 | R18.2 78.99,15.8
N$23
  Top 0.3: U$3.60 20.46,20.46 19.25,19.25 R14.1
N$24
  Top 0.61: BZ1.- 85.85,14.89 T3.3 83.41,16.85 D9.A
N$25
  Top 0.3: U$3.13 28.22,30.72 29.26,31.76 C28.2 29.32,33.51
  Top 0.61: 29.32,33.51 R16.1
N$26
  Top 0.3: 10.53,49.18 T4.1
  Top 0.406: R23.2 9.8,48.63 T4.1 | R24.2 10.53,49.18
N$27
  Top 0.3: 8.22,50.24 T4.3
  Top 0.61: 8.22,50.24 3.81,50.24 IRLED.2
N$28
  Top 0.3: Q2.B 77.5,53.04 | 80.34,53.04 R12.1
  Top 0.508: 80.34,53.04 77.5,53.04 77.5,50.81 R25.2
N$29
  Top 0.508: R25.1 81.25,51.41 T6.3
N$30
  Top 0.3: 85.72,47.68 R26.1 | 88.68,50.46 R36.2
  Top 0.508: 85.72,47.68 T6.1 88.68,50.46
N$31
  Top 0.3: 3.61,44.29 R27.1
  Top 0.61: IRLED.1 3.61,44.29
N$32
  Top 0.3: 28,50.39 R29.1
  Top 0.508: CLED.A 28,50.39
N$34
  Top 0.3: TSOP31236.2 96.89,39.62 | 84.19,42.29 C20.1
  Top 0.61: 95.64,40.87 C19.+ 85.76,40.87 C20.1 | 95.64,40.87 95.89,41.12 TSOP31236.3 | 96.89,39.62 95.64,40.87 | R28.2 84.19,42.29
NRST  (via drill 0.35)
  Top 0.3: 6.86,31.24 R15.1 3.57,28.59 PRG.5 | 6.86,31.24 C12.1 | U$3.7 19.78,27.72 v18.8,28.7 | v8.5,31 7.1,31 6.86,31.24
  Bottom 0.3: v18.8,28.7 10.8,28.7 v8.5,31
OUTTSOP  (via drill 0.35)
  Top 0.3: TSOP31236.1 89.86,37.08 R30.2 85.65,36.85 83,39.5 v26,39.5 | U$3.22 19.96,35.96 v20.5,36.5
  Bottom 0.3: v20.5,36.5 23.5,39.5 v26,39.5
RD  (via drill 0.35)
  Top 0.3: U$3.58 19.46,25.96 v20.3,26.8
  Bottom 0.3: v20.3,26.8 21,27.5 53.5,27.5 55.89,29.89 U$4.7
ROTA  (via drill 0.35)
  Top 0.3: R22.2 C18.1 | C18.1 | 22.48,7.48 v22.5,7.5 | 17.52,7.48 v17.5,7.5 | U$3.45 14.68,26.22 15.7,25.2 v15.7,24.7
  Top 0.406: 22.48,7.48 R22.2 17.52,7.48
  Bottom 0.3: 23.73,7.5 ROTATE.1 | ROTATE.2 16.27,7.5 16.77,7.5 15.78,7.5 15.78,24.73 15.75,24.75 v15.7,24.7
  Bottom 0.406: v22.5,7.5 23.73,7.5 | v17.5,7.5 16.77,7.5
RS  (via drill 0.35)
  Top 0.3: U$3.61 20.96,24.64 v20.9,24.7
  Bottom 0.3: v20.9,24.7 20.9,24.8 21.7,25.6 41.9,25.6 42.9,26.6 54.6,26.6 56.7,28.7 U$4.6
SOUND  (via drill 0.35)
  Top 0.3: U$3.40 11.22,28.72 v10,27.5 | R18.1 72.3,15.8 69.2,12.7 13.3,12.7 v13,13
  Bottom 0.3: v10,27.5 10,16 v13,13
SWCLK  (via drill 0.35)
  Top 0.3: U$3.49 14.96,22.42 14.94,22.4 v14.2,22.4 | PRG.3 2.44,22.4 v11.03,22.4
  Bottom 0.3: v11.03,22.4 v14.2,22.4
SWDIO
  Top 0.3: PRG.4 5.09,24.79 6.02,25.72 U$3.46
UP  (via drill 0.35)
  Top 0.3: 59.98,7.5 R20.2 C13.1 | 62.47,7.47 v62.5,7.5 | U$3.43 15.88,27.22 v16.8,26.3
  Top 0.406: 59.98,7.5 v57.5,7.5 | R20.2 62.47,7.47
  Bottom 0.3: 56.27,7.5 UP.2 51.98,11.3 23.3,11.3 20.8,13.8 20.8,22.3 v16.8,26.3 | 63.73,7.5 UP.1
  Bottom 0.406: v57.5,7.5 56.27,7.5 | v62.5,7.5 63.73,7.5
VCC  (via drill 0.35, 0.6 pad 1.1)
  Top 0.3: C16.1 31,59.49 30.81,59.3 | 34.94,59.49 IC2.3 | 30.81,50.15 30.47,49.81 R29.2 | 22.5,21.5 22.46,21.54 U$3.64 22.46,19.81 C5.2 | U$3.32 14.96,39.78 C8.1 | U$3.19 21.46,37.04 20.47,38.03 C7.2 | v39.7,42.7 39.7,44.06 C21.1 | v60.7,42.9 60.64,42.96 C22.1 | 39.92,9.38 R21.1 | 59.93,9.45 R20.1 | R17.1 | C6.2 12.61,24.72 U$3.48 | 36.93,47 36.5,47 | 79.14,42.5 R28.1 | v80,35 80.05,34.95 | 30.7,45.9 30.57,45.77 30.77,45.97 | v7,20.5 | R15.2 3.57,33.57 | 33.25,37.55 v33.3,37.6 | 19.89,9.5 R22.1 | v32.2,44.3 32.2,44.4
  Top 0.61: 31,59.49 34.94,59.49 | 30.81,50.15 C17.+ 30.81,59.3 | R22.1 39.92,9.38 | R21.1 59.93,9.45 | R20.1 R17.1 | PRG.1 3.65,17.15 v7,20.5 12,15.5 21.5,15.5 23.05,17.05 C5.2 | v7,20.5 C6.2 | 59,47 36.5,47 33.79,47 30.77,50.02 R29.2 30.77,49.52 30.77,45.97 | 59,47 60.64,45.36 C22.1 | C21.1 36.93,47 | 59,47 73,47 v74,46 | v77.5,42.5 79.14,42.5 | 80.05,34.95 R30.1 | 3.57,33.57 v6,36 | C8.1 14.52,42.02 v16,43.5 | C7.2 20.47,42.27 v21.6,43.4 | R16.2 33.25,37.55 | 32.2,44.4 30.7,45.9 | v12.5,9.5 19.89,9.5 | 30.57,45.77 v28.6,43.8
  Bottom 0.3: U$4.27 39.69,42.69 v39.7,42.7 | U$4.1 60.75,42.85 v60.7,42.9
  Bottom 0.61: v74,46 v77.5,42.5 77.5,37.5 v80,35 | v28.6,43.8 28.3,43.5 21.6,43.5 v21.6,43.4 21.5,43.5 v16,43.5 13.5,43.5 6.25,36.25 v6,36 6,21.5 | 6,21.5 v7,20.5 | v33.3,37.6 33.3,43.2 v32.2,44.3 | 6,21.5 6,14.5 11,9.5 v12.5,9.5
VCC/2  (via drill 0.35)
  Top 0.3: 26.36,75.99 R2.2 26.44,76.07 | C2.1 26.87,72.22 | 80.34,54.94 R12.2
  Top 0.508: Q2.E 79,54.94 | 79,54.94 80.34,54.94 | TRAN.P$2 38.28,72.22 44,66.5 44,56 47,53 v71.5,53 | v79,55.5 79,54.94
  Top 0.61: 26.36,75.99 C1.+ 17.49,75.99 15.95,74.45 P1.4 P1.5 | C2.1 26.44,76.07 | 26.87,72.22 TRAN.P$2
  Bottom 0.508: v71.5,53 74,55.5 v79,55.5
VDD  (via drill 0.6 pad 1.1)
  Top 0.3: 5.13,63.11 L1.2 | 7.63,59.45 7.63,59.94 D3.A 7.5,60.16 7.5,59.6 | U$6.1 5.23,61.86 | 19.9,62 19.9,61.08 C4.+ 20.32,60.66 20.48,60.5 20.56,60.58 R3.2 | C15.1 31.12,64.03 | v7,41.5 6.98,41.48
  Top 0.61: U$6.1 5.13,63.11 | 5.23,61.86 7.63,59.45 | C4.+ 16.79,60.7 D7.C 13.6,57.5 10,57.5 | 10,57.5 9.6,57.5 7.5,59.6 | C15.1 28.91,63.91 25.66,60.66 20.32,60.66 | 31.12,64.03 IC2.1 36.97,64.03 38.5,62.5 38.5,54.5 42.5,50.5 67.5,50.5 v68.5,49.5 | BZ1.+ 90.65,21.21 D9.C 78.79,21.21 v73.5,26.5 | 10,57.5 v10,54 | 6.98,41.48 R27.2 | R7.2 87.24,32.3 71.7,32.3 v70,34
  Bottom 0.61: v10,54 10,43.5 8,41.5 v7,41.5 | v68.5,49.5 70,48 v70,34 70,30 v73.5,26.5
WR  (via drill 0.35)
  Top 0.3: U$3.57 18.96,26.76 v19,26.8
  Bottom 0.3: v19,26.8 20.7,28.5 53,28.5 55,30.5 55,39.8 U$4.8

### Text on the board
tPlace: UV LED Controller
tNames: LN-Electronic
